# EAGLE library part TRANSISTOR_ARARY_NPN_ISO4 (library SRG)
NPN Transistor Array 4 isolated transistors Fairchild MMPQ2222A Data Sheet: http://www.fairchildsemi.com/ds/FF/FFB2222A.pdf
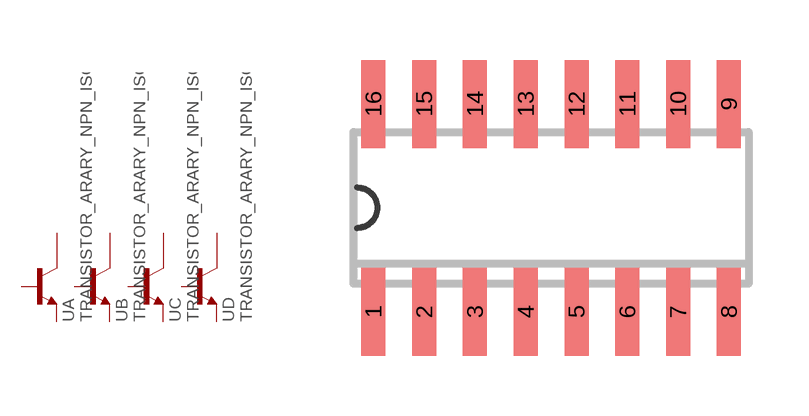
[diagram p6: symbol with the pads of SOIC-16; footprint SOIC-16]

Designator prefix U; gates A=NPN B=NPN C=NPN D=NPN

## TRANSISTOR_ARARY_NPN_ISO4  [SOIC-16]
1  A:COLLECTOR1  pas
2  A:COLLECTOR2  pas
3  B:COLLECTOR1  pas
4  B:COLLECTOR2  pas
5  C:COLLECTOR1  pas
6  C:COLLECTOR2  pas
7  D:COLLECTOR1  pas
8  D:COLLECTOR2  pas
9  D:BASE  pas
10  D:EMITTER  pas
11  C:BASE  pas
12  C:EMITTER  pas
13  B:BASE  pas
14  B:EMITTER  pas
15  A:BASE  pas
16  A:EMITTER  pas

## Footprint SOIC-16 (pad centres in mm)
SOIC-16
smd 0.6 x 2.2: 1 -4.445,-2.6; 2 -3.175,-2.6; 3 -1.905,-2.6; 4 -0.635,-2.6; 5 0.635,-2.6; 6 1.905,-2.6; 7 3.175,-2.6; 8 4.445,-2.6; 9 4.445,2.6; 10 3.175,2.6; 11 1.905,2.6; 12 0.635,2.6; 13 -0.635,2.6; 14 -1.905,2.6; 15 -3.175,2.6; 16 -4.445,2.6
